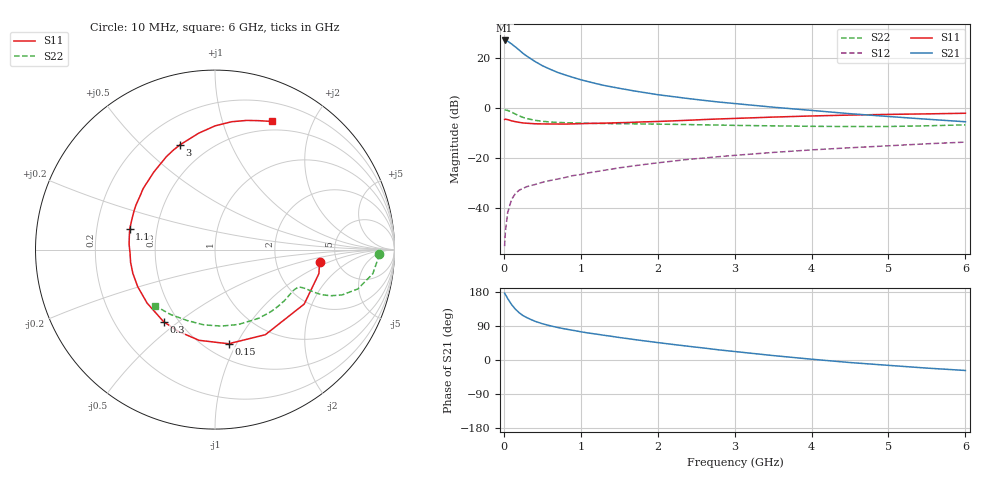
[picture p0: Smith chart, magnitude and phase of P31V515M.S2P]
! SIEMENS Small Signal Semiconductors
! BFP181
! Si NPN RF Bipolar Junction Transistor in SOT143
! VCE = 1.5 V  IC = 15 mA
! Common Emitter S-Parameters:  March  1996
# GHz  S  MA  R  50
!  f  S11  S21  S12  S22
! GHz  MAG  ANG  MAG  ANG  MAG  ANG  MAG  ANG
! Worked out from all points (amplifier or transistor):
!   36 points, 10 MHz to 6 GHz, reference 50 ohm
!   highest |S21| = 27.0 dB at 10 MHz (marker M1)
!   |S21| within 3 dB of that: start of sweep to 165.9 MHz
!   unconditionally stable (mu >= 1): start of sweep to 15.6 MHz; 418.4 MHz to end of sweep
!   at 250 MHz: K = 0.70, MSG = 27.0 dB, |S12| = -32.2 dB
!   at 1.4 GHz: K = 1.67, MAG = 11.7 dB, |S12| = -24.5 dB
!   at 6 GHz: K = 1.32, MAG = 0.7 dB, |S12| = -13.7 dB
!   S11 on the Smith chart (normalised r, x): 10 MHz: 3.68, -0.75; 150 MHz: 0.64, -0.93; 300 MHz: 0.42, -0.44; 1.1 GHz: 0.35, +0.11; 3 GHz: 0.35, +0.66; 6 GHz: 0.40, +1.46
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0.01  0.5868 -6.5  22.45 176.3  0.0017 77.6  0.9144 -1.5
0.02  0.5942 -13.0  22.41 173.0  0.0033 81.1  0.9089 -3.4
0.05  0.5824 -31.4  21.66 162.1  0.008 79.3  0.8894 -8.7
0.1  0.5509 -59.4  19.15 146.5  0.0146 65.5  0.8255 -15.4
0.15  0.53 -81.8  16.65 134.2  0.0193 57.5  0.7523 -19.6
0.2  0.5132 -99.9  14.37 124.6  0.0225 52.9  0.6927 -21.8
0.25  0.4996 -114.2  12.35 117.1  0.0245 49.6  0.6449 -22.9
0.3  0.4933 -125.4  10.87 111.7  0.0265 48.4  0.6108 -23.2
0.4  0.4817 -141.7  8.618 102.5  0.0291 47.4  0.5659 -23.3
0.5  0.4776 -154.3  7.016 95.8  0.0323 46.8  0.54 -23.4
0.6  0.4765 -163.8  5.971 90.4  0.0351 48.3  0.523 -23.7
0.7  0.4756 -171.4  5.135 85.9  0.0376 49.1  0.5119 -24.1
0.8  0.4737 -177.7  4.558 81.8  0.0405 50.2  0.5053 -24.8
1  0.4832 171.1  3.664 74.5  0.0463 51.7  0.4952 -26.8
1.1  0.489 166.3  3.35 71.2  0.0501 52.2  0.4916 -28.0
1.5  0.5054 150.7  2.47 59.4  0.0631 53.2  0.4826 -33.5
2.2  0.5501 128.4  1.683 41.0  0.086 50.9  0.4685 -45.4
3  0.6155 108.4  1.224 22.4  0.1121 46.1  0.4468 -61.3
3.5  0.6548 98.0  1.034 11.7  0.1282 42.8  0.437 -72.7
4.5  0.7187 82.5  0.766 -6.7  0.1591 34.6  0.424 -98.4
5.5  0.7596 71.0  0.594 -21.4  0.1911 26.6  0.4382 -124.4
6  0.7813 66.0  0.528 -27.6  0.2065 21.9  0.4576 -136.9
